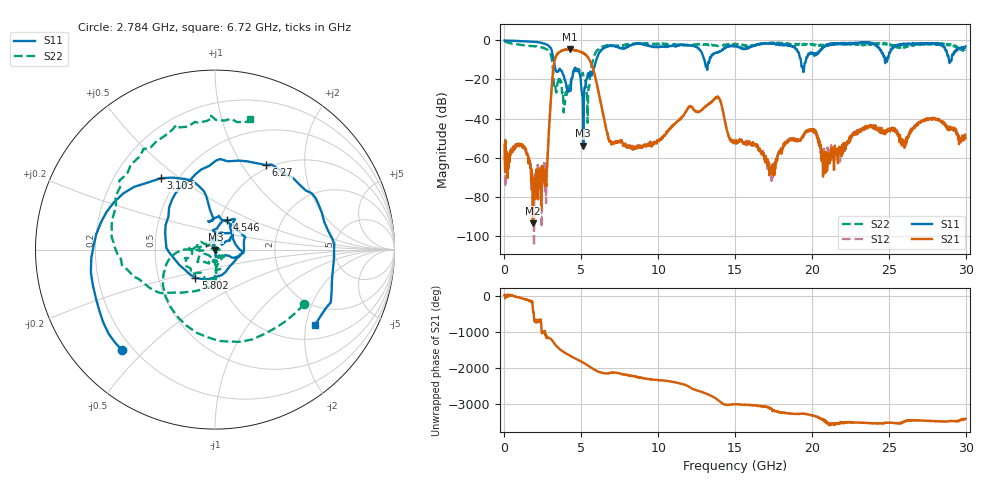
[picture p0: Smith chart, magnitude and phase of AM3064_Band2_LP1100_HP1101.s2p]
# Hz S DB R 50.0
!freq dBS11 angS11 dBS21 angS21 dBS12 angS12 dBS22 angS22
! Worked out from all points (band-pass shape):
!   1600 points, 10 MHz to 29.98 GHz, reference 50 ohm
!   highest |S21| = -4.58 dB at 4.246 GHz (marker M1); lowest = -93.7 dB at 1.847 GHz (marker M2)
!   |S21| within 3 dB of the highest: 3.388 GHz to 5.306 GHz (1.918 GHz wide, 44.1 % of centre)
!   lowest |S11| = -53.9 dB at 5.127 GHz (marker M3), VSWR 1.00, Z = 50.2 - j0.0743 ohm
!   |S11| at or under -10 dB: 3.205 GHz to 5.986 GHz (2.781 GHz wide, 60.5 % of centre); 13.02 GHz to 13.34 GHz (320.3 MHz wide, 2.43 % of centre); 19.27 GHz to 19.61 GHz (336.5 MHz wide, 1.73 % of centre)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
!   |S22| runs from -42.2 to -0.3 dB; largest |S21 - S12| = 0.016
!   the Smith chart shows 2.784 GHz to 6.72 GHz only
!   S11 on the Smith chart (normalised r, x): 2.784 GHz: 0.16, -0.43; 3.103 GHz: 0.41, +0.43; 4.546 GHz: 1.08, +0.37; 5.802 GHz: 0.77, -0.25; 6.27 GHz: 0.95, +1.28; 6.72 GHz: 1.38, -2.26
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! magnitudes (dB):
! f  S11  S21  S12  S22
! 10 MHz  0.0  -53.4  -58.6  -0.3
! 1.191 GHz  -0.4  -53.6  -54.4  -2.4
! 1.847 GHz  -0.7  -93.7  -70.8  -2.9
! 2.784 GHz  -2.3  -63.5  -60.2  -4.7
! 3.103 GHz  -6.0  -20.8  -21.0  -10.9
! 3.403 GHz  -15.9  -7.2  -7.5  -25.6
! 4.246 GHz  -24.6  -4.6  -4.5  -24.4
! 4.546 GHz  -15.0  -5.0  -4.9  -15.1
! 5.015 GHz  -25.4  -6.0  -6.0  -17.9
! 5.127 GHz  -53.9  -6.5  -6.4  -17.9
! 5.408 GHz  -17.9  -8.5  -8.4  -42.2
! 5.802 GHz  -14.4  -15.7  -15.6  -8.5
! 6.27 GHz  -5.2  -32.3  -32.3  -3.8
! 6.72 GHz  -3.1  -47.8  -48.8  -2.5
! 10 GHz  -3.4  -51.3  -51.1  -1.8
! 13.82 GHz  -6.0  -28.9  -29.0  -2.6
! 15 GHz  -2.7  -52.2  -51.9  -1.9
! 17.4 GHz  -1.7  -66.6  -69.7  -1.2
! 19.99 GHz  -6.1  -45.3  -45.9  -1.9
! 20.85 GHz  -3.1  -62.2  -61.0  -2.4
! 25 GHz  -8.1  -45.8  -45.4  -1.7
! 29.98 GHz  -3.1  -50.2  -48.9  -4.8
